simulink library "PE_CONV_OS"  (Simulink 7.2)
settings: Solver=ode45  SolverMode=SingleTasking  StartTime=0.0  StopTime=10.0  RelTol=1e-3
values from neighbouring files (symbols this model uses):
  C = 10e-3*1    (= 0.01)    [INIT_B6_2L_3Ph_IGBT_OS.m]    (also in INIT_B6_3L_3Ph_IGBT_OS.m; INIT_MMC_100L.m = 0.005; INIT_MMC_200L.m = 0.005; INIT_MMC_20L.m)
  FS = 900    [INIT_B6_2L_3Ph_IGBT_OS.m]    (also in INIT_B6_3L_3Ph_IGBT_OS.m; INIT_PWM_2L.m = 1000; INIT_PWM_3L.m = 1000; INIT_PWM_Con.m = 1000)
  LN = 2e-3    (= 0.002)    [INIT_PWM_2L.m]    (also in INIT_PWM_3L.m; INIT_PWM_Con.m; INIT_MMC_100L.m = 0.025; INIT_MMC_200L.m = 0.025)
  LS = 1e-3    (= 0.001)    [INIT_B6_2L_3Ph_IGBT_OS.m]    (also in INIT_B6_3L_3Ph_IGBT_OS.m; INIT_MMC_100L.m = 0.025; INIT_MMC_200L.m = 0.025; INIT_MMC_20L.m = 0.0025)
  LT = LN    (= 0.025)    [INIT_MMC_100L.m]    (also in INIT_MMC_200L.m; INIT_MMC_20L.m = 0.002; INIT_MMC_400L.m)
  Nc = 100    [INIT_MMC_100L.m]    (also in INIT_MMC_200L.m = 200; INIT_MMC_20L.m = 20; INIT_MMC_400L.m = 400)
  NT = sqrt(3)*340/400    [INIT_MMC_100L.m]    (also in INIT_MMC_200L.m; INIT_MMC_20L.m = sqrt(3); INIT_MMC_400L.m)
  Rg = 1e-3    (= 0.001)    [INIT_MMC_100L.m]    (also in INIT_MMC_200L.m; INIT_MMC_20L.m; INIT_MMC_400L.m)
  RN = 0.1    [INIT_PWM_2L.m]    (also in INIT_PWM_3L.m; INIT_PWM_Con.m; INIT_MMC_100L.m; INIT_MMC_200L.m)
  RT = RN    (= 0.1)    [INIT_MMC_100L.m]    (also in INIT_MMC_200L.m; INIT_MMC_20L.m; INIT_MMC_400L.m)
  UC0 = 600    [INIT_B6_2L_3Ph_IGBT_OS.m]    (also in INIT_B6_3L_3Ph_IGBT_OS.m = 500; INIT_MMC_100L.m = 6800; INIT_MMC_200L.m = 3400; INIT_MMC_20L.m = 5000)
undefined symbols (not defined in the file or in its folder): A, DT, FT, L, O1, O2, PHT, T, Td
libraries: simulink_extras x2
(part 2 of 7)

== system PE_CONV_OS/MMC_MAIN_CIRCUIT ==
  MIMC_MC_TDY_SC : S-Function  FunctionName=s_MMC_MC_TDY_SC  Parameters="[LS LN RN LT RT  NT Rg  Ron1  Ron2  Ron3]"  EnableBusSupport=off  mask(MMC_MC_TDY_SC){LS=LS, LN=LN, RN=RN, LT=LT, RT=RT, NT=NT, Rg=Rg, Ron1=1e-3, Ron2=1e-3, Ron3=1e-3}
      mask prompts: LS "LS [H]"; LN "LN [H]"; RN "RN [OHM]"; LT "LT [H]"; RT "RT [OHM]"; Rg "Rg [OHM]"; Ron1 "S1_Ron"; Ron2 "S2_Ron"; Ron3 "S3_Ron"
      mask help: Input Vector: Upper and Lower Arm Voltages =u[0...5] Grid Voltages =u[6...8] DC-Link Current =u[9] Swithing Command for Input Circuit Breaker (Antiparallel Thyristors) =u[10] Swithing Command of Short Circuit Swith (Pos. to Neg. Pass) =u[11] Swithing Command of Short Circuit Swith (Pos. to Ground) =u[12] Swithing Command of Short Circuit Swith (Neg. to Ground) =u[13] Output Vector: Upper and Lower Arm Currents =y[0...5] Converter Currents =y[6...8] Grid Currents =y[9...11] Converter Phase Voltages =y[12...14] DC-Link Voltage=y[15] Parameter Vector: Arm Inductance =p[0] Grid Inductance =p[1] Gr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
  MIMC_MC_TYD_SC : S-Function  FunctionName=s_MMC_MC_TYD_SC  Parameters="[LS LN RN LT RT  NT Rg  Ron1  Ron2  Ron3]"  EnableBusSupport=off  mask(MMC_MC_TYD_SC){LS=LS, LN=LN, RN=RN, LT=LT, RT=RT, NT=NT, Rg=Rg, Ron1=1e-3, Ron2=1e-3, Ron3=1e-3}
      mask prompts: LS "LS [H]"; LN "LN [H]"; RN "RN [OHM]"; LT "LT [H]"; RT "RT [OHM]"; Rg "Rg [OHM]"; Ron1 "S1_Ron"; Ron2 "S2_Ron"; Ron3 "S3_Ron"
      mask help: Input Vector: Upper and Lower Arm Voltages =u[0...5] Grid Voltages =u[6...8] DC-Link Current =u[9] Swithing Command for Input Circuit Breaker (Antiparallel Thyristors) =u[10] Swithing Command of Short Circuit Swith (Pos. to Neg. Pass) =u[11] Swithing Command of Short Circuit Swith (Pos. to Ground) =u[12] Swithing Command of Short Circuit Swith (Neg. to Ground) =u[13] Output Vector: Upper and Lower Arm Currents =y[0...5] Converter Currents =y[6...8] Grid Currents =y[9...11] Converter Phase Voltages =y[12...14] DC-Link Voltage=y[15] Parameter Vector: Arm Inductance =p[0] Grid Inductance =p[1] Gr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
  MIMC_MC_TYY_SC : S-Function  FunctionName=s_MMC_MC_TYY_SC  Parameters="[LS LN RN LT RT  NT Rg  Ron1  Ron2  Ron3]"  EnableBusSupport=off  mask(MMC_MC_TYY_SC){LS=LS, LN=LN, RN=RN, LT=LT, RT=RT, NT=NT, Rg=Rg, Ron1=1e-3, Ron2=1e-3, Ron3=1e-3}
      mask prompts: LS "LS [H]"; LN "LN [H]"; RN "RN [OHM]"; LT "LT [H]"; RT "RT [OHM]"; Rg "Rg [OHM]"; Ron1 "S1_Ron"; Ron2 "S2_Ron"; Ron3 "S3_Ron"
      mask help: Input Vector: Upper and Lower Arm Voltages =u[0...5] Grid Voltages =u[6...8] DC-Link Current =u[9] Swithing Command for Input Circuit Breaker (Antiparallel Thyristors) =u[10] Swithing Command of Short Circuit Swith (Pos. to Neg. Pass) =u[11] Swithing Command of Short Circuit Swith (Pos. to Ground) =u[12] Swithing Command of Short Circuit Swith (Neg. to Ground) =u[13] Output Vector: Upper and Lower Arm Currents =y[0...5] Converter Currents =y[6...8] Grid Currents =y[9...11] Converter Phase Voltages =y[12...14] DC-Link Voltage=y[15] Parameter Vector: Arm Inductance =p[0] Grid Inductance =p[1] Gr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

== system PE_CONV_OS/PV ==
  PV_Array_OS : Subsystem  mask{Isc0=7.9, Ud0=21.8, Ki=1.9e-3, Kv=-0.1, n=1.0, RS=0.28e-3*36, RP=15*36, NC=36, NMs=10, NMp=4, C=1e-3, vC0=0, RL=10000}
      mask prompts: Isc0 "Short Circuit Current at STC Isc0/Module"; Ud0 "Open Circuit Voltage at STC Ud0/Module"; Ki "Short Circuit Current Temp Coeff. Ki/Module"; Kv "Open Circuit Voltage Temp. Coeff. Kv/Module"; n "Diode Idealty Factor n"; RS "Series Resistance Rs/module "RS/Cell*NCells""; RP "Parallel Resistance RP/module "Rp/Cell*NCells""; NC "Number Cells"; NMs "Number Series Modules"; NMp "Number Parallel Modules"; C "Load Capacitor"; vC0 "init Cap Voltage"; RL "Load Res."
      mask help: PV_Array_OS with parameters: N_Cells/Module (NC), N_Series connected Module (NMs) and N_parallel connected Module (NMp) Input Vector u: u[0]=G u[1]=T u[2]=ILd Output Vector y: y[0]=PV.I y[1]=PV.V y[2]=C.I Parameter Vector p: p[0]=Isc0 p[1]=Ud0 p[2]=Ki p[3]=Kv p[4]=n p[5]=RS p[6]=RP p[7]=NC p[8]=NMs p[9]=NMp p[10]=C p[11]=vC0 p[12]=RL You can pause the simulation during running, change the Parameters you want and continue the Simulation
  P_and_O : Subsystem  mask{DeltaD=0.0001}
      mask help: MPPT controller based on the Perturb & Observe algorithm. D output = Duty cycle of the boost converter (value between 0 and 1) DeltaD = 0.0001; Increment value used to increase/decrease the duty cycle D

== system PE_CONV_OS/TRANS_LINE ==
  TL-DIST-PAR-OS : Subsystem  mask(1-Phase TL-N-DIST-PAR){L=1.3e-3, C=8.9e-9, R=0.05, TL=200, RS=50}
      mask prompts: L "L/km"; C "C/km"; R "R/km"; TL "Length[km]"
      mask help: 1 Phase frequency independent trans. Line based on the Bergerons model. Input Vector: u[0]=Input Voltage u[1]=Load Current Output Vector: y[0]=Input Voltage y[1]=Output Voltage y[2]=Input Current y[3]=Output Current PArameter Vector: p[0]= TL-Inductane L/km p[1]= TL-Capacitance C/km p[2]= TL-Resistance R/km p[3]= TL-Length [km] p[4]= TL-Input Resistance R
  TL-N-PI-3PH : Subsystem  mask(3-Phase TL N-PI-Sections){R=0.01273, L=0.9337e-3, C=12.74e-9, TL=100, N=5, RS=1, LS=1e-3}
      mask prompts: R "R/km"; L "L/km"; C "C/km"; TL "Length[km]"; N "N_Sections"
      mask help: 3 Phase trans. Line as N-PI-Sections Input Vector: u[0,1,2]=Input Voltages u[3.4]=Load Currents Output Vector: y[0,1,2]=Input Currents y[3,4,5]=Output Currents y[6,7,8]=Input Voltages y[9,10,11]=Output Voltages PArameter Vector: p[0]= TL-Resistance R/km p[1]= TL-Inductane L/km p[2]= TL-Capacitance C/km p[3]= TL-Length [km] p[4]= Number of PI-Sections N p[5]= Source-Input Resistance R
  TL-SEQ-3PH : Subsystem  mask(3-Phase TL N-Sections){R1=0.01273, R0=0.3864, L1=0.9337e-3, L0=4.1264e-3, C1=12.74e-9, C0=7.751e-9, TL=100, NS=5, RS=1, LS=1e-3}
      mask prompts: R1 "R1/km"; R0 "R0/km"; L1 "L1/km"; L0 "L0/km"; C1 "C1/km"; C0 "C0/km"; TL "Length[km]"; NS "N-Sections"
      mask help: 3 Phase trans. Line Parameters are entered as Positive and Zero Sequence Parameters Input Vector: u[0,1,2]=Input Voltages u[3,4]=Load Currents Output Vector: y[0,1,2]=Input Currents y[3,4,5]=Output Currents y[6,7,8]=Input Voltages y[9,10,11]=Output Voltages PArameter Vector: p[0]= TL-Pos. Seq. Resistance R1/km p[1]= TL-Zero Seq. Resistance R0/km p[2]= TL-Pos. Seq. Inductance L1/km p[3]= TL-Zero Seq. Inductance L0/km p[4]= TL-Pos. Seq. Capacitance C1/km p[5]= TL-Zero Seq. Capacitance C0/km p[6]= TL-Length [km] p[7]= TL-N-Sections p[8]= Source-Input Resistance RS p[9]= Source-Input Inductance LS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
  TL_N-PI_1PH : Subsystem  mask(1-Phase TL N-PI-Sections){L=1.3e-3, C=8.9e-9, R=0.05, TL=200, N=100, R1=50}
      mask prompts: L "L/km"; C "C/km"; R "R/km"; TL "Length[km]"; N "N_Sections"
      mask help: 1 Phase trans. Line as N-PI-Sections Input Vector: u[0]=Input Voltage u[1]=Load Current Output Vector: y[0]=Input Voltage y[1]=Output Voltage y[2]=Input Current y[3]=Output Current PArameter Vector: p[0]= TL-Inductane L/km p[1]= TL-Capacitance C/km p[2]= TL-Resistance R/km p[3]= TL-Length [km] p[4]= Number of PI-Sections N p[5]= TL-Input Resistance R

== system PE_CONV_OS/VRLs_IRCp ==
  IS_IRCp : Subsystem  mask(IRCp_OS){R=100, C=100e-6, VC0=0, RCs=1e-6}
      mask prompts: R "Res"; C "Cap"; VC0 "Initial Cap Voltage"; RCs "Cap Res"
      mask help: Open source IRC_Parallel Input Vector: u[0]= Is, Source Current u[1]= IL, Load Current Output Vector: y[0]=IC, Capacitance current y[1]=VC, Capacitance Voltage y[2]=VR, Resistance Voltage Parameter Vector: p[0]=R p[1]=C p[2]=VC0
  IS_IRCp_3PH : Subsystem  mask(IRCp_3PH_OS){R=100, C=100e-6, RCs=1e-6}
      mask prompts: R "Output Resistance"; C "Output Capacitance"
      mask help: Open source 3 Phase IRC_Parallel u[0,1,2]= Is1, Is2, Is3, Source Current u[3,4,5]= IL1, IL2, IL3, Load Current Output Vector: y[0,1,2]=IC_123 y[3,4,5]=VC_123 y[6,7,8]=IR_123 Parameter Vector: p[0]=R p[1]=C p[2]=RCs
  IS_VRLs : Subsystem  mask(VRLs_OS){R=1, L=10e-3, IL0=0, RLp=1e6}
      mask prompts: R "Output Resistance"; L "Output Inductance"; IL0 "Initial Inductor Current"; RLp "Ind. Parallel Res"
      mask help: Open source VRL_Series Input Vector: u[0]= Vs, Source Voltage u[1]= E, Load Voltage Output Vector: y[0]=IL, Load current y[1]=VL, Inductance Voltage y[2]=VR, Resistance Voltage Parameter Vector: p[0]=R p[1]=L p[2]=IL0 p[3]=RLp
  IS_VRLs_3PH : Subsystem  mask(VRLs_3PH_OS){R=1, L=1e-3, RLp=1e6}
      mask prompts: R "Output Resistance"; L "Output Inductance"; RLp "Ind. Parallel Res"
      mask help: Open source 3 Phase VRL_Series Input Vector: u[0,1,2]= Is1, Is2, Is3, Source Currents u[3,4,5]= E1, E2, E3, Load Voltages Output Vector: y[0,1,2]=IL1, IL2, IL3 Inductance currents y[3,4,5]=VL1, VL2, VL3 Inductance Voltages y[6,7,8]=VR1, VR2, VR3 Resistance Voltages Parameter Vector: p[0]=R p[1]=L
  VS_IRLs : Subsystem  mask(IRCp_OS){R=100}
      mask prompts: R "Res"
      mask help: Open source IRC_Parallel Input Vector: u[0]= Is, Source Current u[1]= IL, Load Current Output Vector: y[0]=IL, Load current y[1]=VL, Load Voltage Parameter Vector: p[0]=R
  VS_IRLs_3PH : Subsystem  mask(IRCp_3PH_OS){R=100}
      mask prompts: R "Output Resistance"
      mask help: Open source 3 Phase IRC_Parallel u[0,1,2]= Is1, Is2, Is3, Source Current u[3,4,5]= IL1, IL2, IL3, Load Current Output Vector: y[0,1,2]=IL_123 y[3,4,5]=VL_123 Parameter Vector: p[0]=R
  VS_VRLs : Subsystem  mask(VRLs_OS){R=1, L=10e-3, IL0=0, RLp=1e6}
      mask prompts: R "Output Resistance"; L "Output Inductance"; IL0 "Initial Inductor Current"; RLp "Ind. Parallel Res"
      mask help: Open source VRL_Series Input Vector: u[0]= Vs, Source Voltage u[1]= E, Load Voltage Output Vector: y[0]=IL, Load current y[1]=VL, Inductance Voltage y[2]=VR, Resistance Voltage Parameter Vector: p[0]=R p[1]=L p[2]=IL0
  VS_VRLs_3PH : Subsystem  mask(VRLs_3PH_OS){R=1, L=1e-3, RLp=1e6}
      mask prompts: R "Output Resistance"; L "Output Inductance"; RLp "Ind. Parallel Res"
      mask help: Open source 3 Phase VRL_Series Input Vector: u[0,1,2]= Vs1, Vs2, Vs3, Source Voltages u[3,4,5]= E1, E2, E3, Load Voltages Output Vector: y[0,1,2]=IL1, IL2, IL3 Load currents y[3,4,5]=VL1, VL2, VL3 Inductance Voltages Parameter Vector: p[0]=R p[1]=L

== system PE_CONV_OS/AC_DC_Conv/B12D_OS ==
  vS : Inport  OutDataType=sfix(16)  OutScaling=2^0
  iDC1 : Inport  Port=2  OutDataType=sfix(16)  OutScaling=2^0
  iDC2 : Inport  Port=3  OutDataType=sfix(16)  OutScaling=2^0
  Mux : Mux  Inputs="[3  1  1]"
  b12d : S-Function  FunctionName=s_b12d_OS  Parameters="[ LS  nyy  nyd   LT  LD ILD0 C  VC0  RL]"  EnableBusSupport=off
  "iD1, vD1" : Outport  OutDataType=sfix(16)  OutScaling=2^0
  "iD2, vD2" : Outport  Port=2  OutDataType=sfix(16)  OutScaling=2^0
  "iLc1, iLc2, iLc3" : Outport  Port=3  OutDataType=sfix(16)  OutScaling=2^0
  iLd1,iLd2 : Outport  Port=4  OutDataType=sfix(16)  OutScaling=2^0
  vDC1,vDC2 : Outport  Port=5  OutDataType=sfix(16)  OutScaling=2^0
  vC1,vC2 : Outport  Port=6  OutDataType=sfix(16)  OutScaling=2^0
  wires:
  b12d/6 -> vC1,vC2/1
  b12d/5 -> vDC1,vDC2/1
  iDC2/1 -> Mux/3
  b12d/3 -> "iLc1, iLc2, iLc3"/1
  b12d/1 -> "iD1, vD1"/1
  b12d/2 -> "iD2, vD2"/1
  vS/1 -> Mux/1
  iDC1/1 -> Mux/2
  Mux/1 -> b12d/1
  b12d/4 -> iLd1,iLd2/1

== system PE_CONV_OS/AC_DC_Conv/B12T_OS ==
  SWs : Inport  OutDataType=sfix(16)  OutScaling=2^0
  SWs1 : Inport  Port=2  OutDataType=sfix(16)  OutScaling=2^0
  vS : Inport  Port=3  OutDataType=sfix(16)  OutScaling=2^0
  iDC1 : Inport  Port=4  OutDataType=sfix(16)  OutScaling=2^0
  iDC2 : Inport  Port=5  OutDataType=sfix(16)  OutScaling=2^0
  Mux : Mux  Inputs="[6   6   3  1  1]"
  b12t : S-Function  FunctionName=s_b12t_OS  Parameters="[LS  LT1 LT2  LD ILD0  C  VC0 RL]"  EnableBusSupport=off
  i1T1;v1T! : Outport  OutDataType=sfix(16)  OutScaling=2^0
  i2T1,i2T1 : Outport  Port=2  OutDataType=sfix(16)  OutScaling=2^0
  "iL1, iL2, iL3" : Outport  Port=3  OutDataType=sfix(16)  OutScaling=2^0
  iDC1,iDC2 : Outport  Port=4  OutDataType=sfix(16)  OutScaling=2^0
  vDC1,vDC1 : Outport  Port=5  OutDataType=sfix(16)  OutScaling=2^0
  vC1,vC2 : Outport  Port=6  OutDataType=sfix(16)  OutScaling=2^0
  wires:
  b12t/6 -> vC1,vC2/1
  b12t/5 -> vDC1,vDC1/1
  b12t/4 -> iDC1,iDC2/1
  b12t/3 -> "iL1, iL2, iL3"/1
  iDC2/1 -> Mux/5
  SWs1/1 -> Mux/2
  SWs/1 -> Mux/1
  vS/1 -> Mux/3
  b12t/1 -> i1T1;v1T!/1
  b12t/2 -> i2T1,i2T1/1
  iDC1/1 -> Mux/4
  Mux/1 -> b12t/1

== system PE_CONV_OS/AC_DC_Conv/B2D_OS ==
  vS : Inport  OutDataType=sfix(16)  OutScaling=2^0
  iDC : Inport  Port=2  OutDataType=sfix(16)  OutScaling=2^0
  Mux : Mux  Inputs=2
  b6d : S-Function  FunctionName=s_b2d_OS  Parameters="[ LS LD  ILD0  C  VC0 RD]"  EnableBusSupport=off
  iD1,vD1 : Outport  OutDataType=sfix(16)  OutScaling=2^0
  iLc : Outport  Port=2  OutDataType=sfix(16)  OutScaling=2^0
  iLd : Outport  Port=3  OutDataType=sfix(16)  OutScaling=2^0
  vDC : Outport  Port=4  OutDataType=sfix(16)  OutScaling=2^0
  vC : Outport  Port=5  OutDataType=sfix(16)  OutScaling=2^0
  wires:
  b6d/5 -> vC/1
  b6d/4 -> vDC/1
  b6d/3 -> iLd/1
  Mux/1 -> b6d/1
  iDC/1 -> Mux/2
  vS/1 -> Mux/1
  b6d/2 -> iLc/1
  b6d/1 -> iD1,vD1/1

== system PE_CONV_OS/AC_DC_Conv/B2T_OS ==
  SWs : Inport  OutDataType=sfix(16)  OutScaling=2^0
  vS : Inport  Port=2  OutDataType=sfix(16)  OutScaling=2^0
  iDC : Inport  Port=3  OutDataType=sfix(16)  OutScaling=2^0
  Mux : Mux  Inputs="[2 1  1]"
  b6d : S-Function  FunctionName=s_b2t_OS  Parameters="[ LS LD ILD0 C  VC0 RL]"  EnableBusSupport=off
  iT1,vT1 : Outport  OutDataType=sfix(16)  OutScaling=2^0
  Ilc : Outport  Port=2  OutDataType=sfix(16)  OutScaling=2^0
  iLd : Outport  Port=3  OutDataType=sfix(16)  OutScaling=2^0
  vDC : Outport  Port=4  OutDataType=sfix(16)  OutScaling=2^0
  vC : Outport  Port=5  OutDataType=sfix(16)  OutScaling=2^0
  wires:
  b6d/5 -> vC/1
  SWs/1 -> Mux/1
  vS/1 -> Mux/2
  b6d/1 -> iT1,vT1/1
  b6d/2 -> Ilc/1
  b6d/3 -> iLd/1
  iDC/1 -> Mux/3
  Mux/1 -> b6d/1
  b6d/4 -> vDC/1

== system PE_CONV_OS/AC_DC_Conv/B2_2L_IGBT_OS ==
  SWs : Inport  OutDataType=sfix(16)  OutScaling=2^0
  vS : Inport  Port=2  OutDataType=sfix(16)  OutScaling=2^0
  iDC : Inport  Port=3  OutDataType=sfix(16)  OutScaling=2^0
  Mux : Mux  Inputs="[4  1  1]"
  b2_2L_IGBT : S-Function  FunctionName=s_b2_2L_IGBT_OS  Parameters="[ LS  C  VC0 RL]"  EnableBusSupport=off
  iT1,iD1,vT1 : Outport  OutDataType=sfix(16)  OutScaling=2^0
  iT2,iD2,vT2 : Outport  Port=2  OutDataType=sfix(16)  OutScaling=2^0
  iLs : Outport  Port=3  OutDataType=sfix(16)  OutScaling=2^0
  vDC : Outport  Port=4  OutDataType=sfix(16)  OutScaling=2^0
  va : Outport  Port=5  OutDataType=sfix(16)  OutScaling=2^0
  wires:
  b2_2L_IGBT/4 -> vDC/1
  Mux/1 -> b2_2L_IGBT/1
  iDC/1 -> Mux/3
  b2_2L_IGBT/3 -> iLs/1
  b2_2L_IGBT/2 -> iT2,iD2,vT2/1
  b2_2L_IGBT/1 -> iT1,iD1,vT1/1
  vS/1 -> Mux/2
  SWs/1 -> Mux/1
  b2_2L_IGBT/5 -> va/1

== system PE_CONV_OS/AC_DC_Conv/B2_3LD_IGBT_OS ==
  SWs : Inport  OutDataType=sfix(16)  OutScaling=2^0
  vS : Inport  Port=2  OutDataType=sfix(16)  OutScaling=2^0
  iDC : Inport  Port=3  OutDataType=sfix(16)  OutScaling=2^0
  Mux : Mux  Inputs="[8  1  1]"
  b2_2L_IGBT : S-Function  FunctionName=s_b2_3LD_IGBT_OS  Parameters="[ LS  C  VC0 RL]"  EnableBusSupport=off
  iT1,iD1,vT1 : Outport  OutDataType=sfix(16)  OutScaling=2^0
  iT2,iD2,vT2 : Outport  Port=2  OutDataType=sfix(16)  OutScaling=2^0
  iLs : Outport  Port=3  OutDataType=sfix(16)  OutScaling=2^0
  vDC12 : Outport  Port=4  OutDataType=sfix(16)  OutScaling=2^0
  va : Outport  Port=5  OutDataType=sfix(16)  OutScaling=2^0
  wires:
  b2_2L_IGBT/5 -> va/1
  SWs/1 -> Mux/1
  vS/1 -> Mux/2
  b2_2L_IGBT/1 -> iT1,iD1,vT1/1
  b2_2L_IGBT/2 -> iT2,iD2,vT2/1
  b2_2L_IGBT/3 -> iLs/1
  iDC/1 -> Mux/3
  Mux/1 -> b2_2L_IGBT/1
  b2_2L_IGBT/4 -> vDC12/1

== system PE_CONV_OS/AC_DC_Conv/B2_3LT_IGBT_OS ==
  SWs : Inport  OutDataType=sfix(16)  OutScaling=2^0
  vS : Inport  Port=2  OutDataType=sfix(16)  OutScaling=2^0
  iDC : Inport  Port=3  OutDataType=sfix(16)  OutScaling=2^0
  Mux : Mux  Inputs="[8  1  1]"
  b2_2L_IGBT : S-Function  FunctionName=s_b2_3LT_IGBT_OS  Parameters="[ LS  C  VC0 RL]"  EnableBusSupport=off
  iT1,iD1,vT1 : Outport  OutDataType=sfix(16)  OutScaling=2^0
  iT2,iD2,vT2 : Outport  Port=2  OutDataType=sfix(16)  OutScaling=2^0
  iLs : Outport  Port=3  OutDataType=sfix(16)  OutScaling=2^0
  vDC1,vDC2 : Outport  Port=4  OutDataType=sfix(16)  OutScaling=2^0
  va : Outport  Port=5  OutDataType=sfix(16)  OutScaling=2^0
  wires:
  b2_2L_IGBT/4 -> vDC1,vDC2/1
  Mux/1 -> b2_2L_IGBT/1
  iDC/1 -> Mux/3
  b2_2L_IGBT/3 -> iLs/1
  b2_2L_IGBT/2 -> iT2,iD2,vT2/1
  b2_2L_IGBT/1 -> iT1,iD1,vT1/1
  vS/1 -> Mux/2
  SWs/1 -> Mux/1
  b2_2L_IGBT/5 -> va/1

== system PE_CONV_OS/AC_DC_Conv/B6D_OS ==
  vS : Inport  OutDataType=sfix(16)  OutScaling=2^0
  iDC : Inport  Port=2  OutDataType=sfix(16)  OutScaling=2^0
  Mux : Mux  Inputs=2
  b6d : S-Function  FunctionName=s_b6d_OS  Parameters="[ LS  LD ILD0  C  VC0 RL]"  EnableBusSupport=off
  iD1,vD1 : Outport  OutDataType=sfix(16)  OutScaling=2^0
  "iLc1, iLc2, iLc3" : Outport  Port=2  OutDataType=sfix(16)  OutScaling=2^0
  iLd : Outport  Port=3  OutDataType=sfix(16)  OutScaling=2^0
  vDC : Outport  Port=4  OutDataType=sfix(16)  OutScaling=2^0
  vC : Outport  Port=5  OutDataType=sfix(16)  OutScaling=2^0
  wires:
  b6d/5 -> vC/1
  b6d/3 -> iLd/1
  b6d/2 -> "iLc1, iLc2, iLc3"/1
  b6d/4 -> vDC/1
  Mux/1 -> b6d/1
  iDC/1 -> Mux/2
  vS/1 -> Mux/1
  b6d/1 -> iD1,vD1/1

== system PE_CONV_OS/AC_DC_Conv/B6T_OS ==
  SWs : Inport  OutDataType=sfix(16)  OutScaling=2^0
  vS : Inport  Port=2  OutDataType=sfix(16)  OutScaling=2^0
  iDC : Inport  Port=3  OutDataType=sfix(16)  OutScaling=2^0
  Mux : Mux  Inputs="[6 3  1]"
  b6d : S-Function  FunctionName=s_b6t_OS  Parameters="[ LS  LD ILD0 C  VC0 RL]"  EnableBusSupport=off
  iT1,vT1 : Outport  OutDataType=sfix(16)  OutScaling=2^0
  "iLc1, iLc2, iLc3" : Outport  Port=2  OutDataType=sfix(16)  OutScaling=2^0
  iDC1 : Outport  Port=3  OutDataType=sfix(16)  OutScaling=2^0
  vDC : Outport  Port=4  OutDataType=sfix(16)  OutScaling=2^0
  vC : Outport  Port=5  OutDataType=sfix(16)  OutScaling=2^0
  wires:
  b6d/5 -> vC/1
  SWs/1 -> Mux/1
  vS/1 -> Mux/2
  b6d/1 -> iT1,vT1/1
  b6d/2 -> "iLc1, iLc2, iLc3"/1
  b6d/3 -> iDC1/1
  iDC/1 -> Mux/3
  Mux/1 -> b6d/1
  b6d/4 -> vDC/1

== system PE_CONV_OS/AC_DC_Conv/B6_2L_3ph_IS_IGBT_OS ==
  SWs : Inport  OutDataType=sfix(16)  OutScaling=2^0
  IS : Inport  Port=2  OutDataType=sfix(16)  OutScaling=2^0
  iDC : Inport  Port=3  OutDataType=sfix(16)  OutScaling=2^0
  Mux : Mux  Inputs="[6  3  1]"
  b2_IGBT : S-Function  FunctionName=s_b6_2L_3Ph_IS_IGBT_OS  Parameters="[C  UC0 RL]"  EnableBusSupport=off
  iT1,iD1,vT1 : Outport  OutDataType=sfix(16)  OutScaling=2^0
  iT2,iD2,vT2 : Outport  Port=2  OutDataType=sfix(16)  OutScaling=2^0
  vDC : Outport  Port=3  OutDataType=sfix(16)  OutScaling=2^0
  vabc : Outport  Port=4  OutDataType=sfix(16)  OutScaling=2^0
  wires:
  b2_IGBT/5 -> vabc/1
  SWs/1 -> Mux/1
  IS/1 -> Mux/2
  b2_IGBT/1 -> iT1,iD1,vT1/1
  b2_IGBT/2 -> iT2,iD2,vT2/1
  iDC/1 -> Mux/3
  Mux/1 -> b2_IGBT/1
  b2_IGBT/4 -> vDC/1

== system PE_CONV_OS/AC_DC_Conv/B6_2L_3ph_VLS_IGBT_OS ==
  SWs : Inport  OutDataType=sfix(16)  OutScaling=2^0
  vS : Inport  Port=2  OutDataType=sfix(16)  OutScaling=2^0
  iDC : Inport  Port=3  OutDataType=sfix(16)  OutScaling=2^0
  Mux : Mux  Inputs="[6  3  1]"
  b2_IGBT : S-Function  FunctionName=s_b6_2L_3Ph_VLS_IGBT_OS  Parameters="[ LS  C  UC0 RL]"  EnableBusSupport=off
  iT1,iD1,vT1 : Outport  OutDataType=sfix(16)  OutScaling=2^0
  iT2,iD2,vT2 : Outport  Port=2  OutDataType=sfix(16)  OutScaling=2^0
  iLs : Outport  Port=3  OutDataType=sfix(16)  OutScaling=2^0
  vDC : Outport  Port=4  OutDataType=sfix(16)  OutScaling=2^0
  vabc : Outport  Port=5  OutDataType=sfix(16)  OutScaling=2^0
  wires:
  b2_IGBT/4 -> vDC/1
  Mux/1 -> b2_IGBT/1
  iDC/1 -> Mux/3
  b2_IGBT/3 -> iLs/1
  b2_IGBT/2 -> iT2,iD2,vT2/1
  b2_IGBT/1 -> iT1,iD1,vT1/1
  vS/1 -> Mux/2
  SWs/1 -> Mux/1
  b2_IGBT/5 -> vabc/1

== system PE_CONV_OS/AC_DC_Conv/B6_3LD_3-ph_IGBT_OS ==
  SWs : Inport  OutDataType=sfix(16)  OutScaling=2^0
  vS : Inport  Port=2  OutDataType=sfix(16)  OutScaling=2^0
  iDC : Inport  Port=3  OutDataType=sfix(16)  OutScaling=2^0
  Mux : Mux  Inputs="[12  3  1]"
  b2_IGBT : S-Function  FunctionName=s_b6_3LD_3Ph_IGBT_OS  Parameters="[ LS  C  VC0 RL]"  EnableBusSupport=off
  iT1,iD1,vT1 : Outport  OutDataType=sfix(16)  OutScaling=2^0
  iT2,iD2,vT2 : Outport  Port=2  OutDataType=sfix(16)  OutScaling=2^0
  iLs : Outport  Port=3  OutDataType=sfix(16)  OutScaling=2^0
  vDC : Outport  Port=4  OutDataType=sfix(16)  OutScaling=2^0
  vab : Outport  Port=5  OutDataType=sfix(16)  OutScaling=2^0
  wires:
  b2_IGBT/5 -> vab/1
  SWs/1 -> Mux/1
  vS/1 -> Mux/2
  b2_IGBT/1 -> iT1,iD1,vT1/1
  b2_IGBT/2 -> iT2,iD2,vT2/1
  b2_IGBT/3 -> iLs/1
  iDC/1 -> Mux/3
  Mux/1 -> b2_IGBT/1
  b2_IGBT/4 -> vDC/1

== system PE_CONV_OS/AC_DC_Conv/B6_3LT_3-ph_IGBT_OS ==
  SWs : Inport  OutDataType=sfix(16)  OutScaling=2^0
  vS : Inport  Port=2  OutDataType=sfix(16)  OutScaling=2^0
  iDC : Inport  Port=3  OutDataType=sfix(16)  OutScaling=2^0
  Mux : Mux  Inputs="[12  3  1]"
  b2_IGBT : S-Function  FunctionName=s_b6_3LT_3Ph_IGBT_OS  Parameters="[ LS  C  VC0 RL]"  EnableBusSupport=off
  iT1,iD1,vT1 : Outport  OutDataType=sfix(16)  OutScaling=2^0
  iT2,iD2,vT2 : Outport  Port=2  OutDataType=sfix(16)  OutScaling=2^0
  iLs123 : Outport  Port=3  OutDataType=sfix(16)  OutScaling=2^0
  vDC12 : Outport  Port=4  OutDataType=sfix(16)  OutScaling=2^0
  vab : Outport  Port=5  OutDataType=sfix(16)  OutScaling=2^0
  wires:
  b2_IGBT/4 -> vDC12/1
  Mux/1 -> b2_IGBT/1
  iDC/1 -> Mux/3
  b2_IGBT/3 -> iLs123/1
  b2_IGBT/2 -> iT2,iD2,vT2/1
  b2_IGBT/1 -> iT1,iD1,vT1/1
  vS/1 -> Mux/2
  SWs/1 -> Mux/1
  b2_IGBT/5 -> vab/1

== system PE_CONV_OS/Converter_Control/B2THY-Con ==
  In1 : Inport  OutDataType=sfix(16)  OutScaling=2^0
  Mux : Mux
  THY-Con : Subsystem  mask(THY-Con){F=F, PH=PH, TD=TD}
      mask prompts: F "Frequency"; PH "Phase Angle (Degree)"; TD "Puls Duration"
      mask init:
      | x=0:pi/20:2*pi;
      | y=cos(x);
  THY-Con1 : Subsystem  mask(THY-Con){F=F, PH=-PH, TD=TD}
      mask prompts: F "Frequency"; PH "Phase Angle (Degree)"; TD "Puls Duration"
      mask init:
      | x=0:pi/20:2*pi;
      | y=cos(x);
  Out1 : Outport
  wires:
  In1/1 -> THY-Con/1(In1), THY-Con1/1(In1)
  THY-Con/1(Out1) -> Mux/1, Mux/4
  THY-Con1/1(Out1) -> Mux/2, Mux/3
  Mux/1 -> Out1/1

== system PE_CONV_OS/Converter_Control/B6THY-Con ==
  In1 : Inport  OutDataType=sfix(16)  OutScaling=2^0
  DT1 : DataTypeConversion
  Mux : Mux  Inputs=6
  OR{,1..5} (6 alike) : Logic  Operator=OR
  THY-Con : Subsystem  mask(THY-Con){F=F, PH=PH, TD=TD}
      mask prompts: F "Frequency"; PH "Phase Angle (Degree)"; TD "Puls Duration"
      mask init:
      | x=0:pi/20:2*pi;
      | y=cos(x);
  THY-Con1 : Subsystem  mask(THY-Con){F=F, PH=PH-60, TD=TD}
      mask prompts: F "Frequency"; PH "Phase Angle (Degree)"; TD "Puls Duration"
      mask init:
      | x=0:pi/20:2*pi;
      | y=cos(x);
  THY-Con2 : Subsystem  mask(THY-Con){F=F, PH=PH-120, TD=TD}
      mask prompts: F "Frequency"; PH "Phase Angle (Degree)"; TD "Puls Duration"
      mask init:
      | x=0:pi/20:2*pi;
      | y=cos(x);
  THY-Con3 : Subsystem  mask(THY-Con){F=F, PH=PH-180, TD=TD}
      mask prompts: F "Frequency"; PH "Phase Angle (Degree)"; TD "Puls Duration"
      mask init:
      | x=0:pi/20:2*pi;
      | y=cos(x);
  THY-Con4 : Subsystem  mask(THY-Con){F=F, PH=PH-240, TD=TD}
      mask prompts: F "Frequency"; PH "Phase Angle (Degree)"; TD "Puls Duration"
      mask init:
      | x=0:pi/20:2*pi;
      | y=cos(x);
  THY-Con5 : Subsystem  mask(THY-Con){F=F, PH=PH-300, TD=TD}
      mask prompts: F "Frequency"; PH "Phase Angle (Degree)"; TD "Puls Duration"
      mask init:
      | x=0:pi/20:2*pi;
      | y=cos(x);
  Out1 : Outport
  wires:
  OR5/1 -> Mux/6
  OR4/1 -> Mux/5
  OR3/1 -> Mux/4
  OR2/1 -> Mux/3
  OR1/1 -> Mux/2
  OR/1 -> Mux/1
  THY-Con/1(Out1) -> OR5/2, OR/1
  THY-Con5/1(Out1) -> OR4/2, OR5/1
  THY-Con4/1(Out1) -> OR3/2, OR4/1
  THY-Con3/1(Out1) -> OR2/2, OR3/1
  THY-Con2/1(Out1) -> OR1/2, OR2/1
  THY-Con1/1(Out1) -> OR/2, OR1/1
  Mux/1 -> DT1/1
  In1/1 -> THY-Con4/1(In1), THY-Con5/1(In1), THY-Con3/1(In1), THY-Con2/1(In1), THY-Con1/1(In1), THY-Con/1(In1)
  DT1/1 -> Out1/1

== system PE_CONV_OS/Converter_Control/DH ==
  I : Inport  OutDataType=sfix(16)  OutScaling=2^0
  Gain : Gain  Gain=1/2  ParameterDataType=sfix(16)  ParameterScaling=2^0  OutDataType=sfix(16)  OutScaling=2^0
  MinMax : MinMax  OutDataType=sfix(16)  OutScaling=2^0
  MinMax1 : MinMax  Function=max  OutDataType=sfix(16)  OutScaling=2^0
  Sum6 : Sum  Inputs=--  OutDataType=sfix(16)  OutScaling=2^0
  Sum7 : Sum  OutDataType=sfix(16)  OutScaling=2^0
  O : Outport  InitialOutput=0
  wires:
  I/1 -> MinMax1/1, MinMax/1, Sum7/1
  MinMax/1 -> Sum6/1
  MinMax1/1 -> Sum6/2
  Sum6/1 -> Gain/1
  Gain/1 -> Sum7/2
  Sum7/1 -> O/1

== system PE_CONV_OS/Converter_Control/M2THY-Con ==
  In1 : Inport  OutDataType=sfix(16)  OutScaling=2^0
  Mux : Mux  Inputs=2
  THY-Con : Subsystem  mask(THY-Con){F=F, PH=PH, TD=TD}
      mask prompts: F "Frequency"; PH "Phase Angle (Degree)"; TD "Puls Duration"
      mask init:
      | x=0:pi/20:2*pi;
      | y=cos(x);
  THY-Con1 : Subsystem  mask(THY-Con){F=F, PH=-PH, TD=TD}
      mask prompts: F "Frequency"; PH "Phase Angle (Degree)"; TD "Puls Duration"
      mask init:
      | x=0:pi/20:2*pi;
      | y=cos(x);
  Out1 : Outport
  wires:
  Mux/1 -> Out1/1
  THY-Con/1(Out1) -> Mux/1
  THY-Con1/1(Out1) -> Mux/2
  In1/1 -> THY-Con/1(In1), THY-Con1/1(In1)

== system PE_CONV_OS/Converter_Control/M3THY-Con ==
  In1 : Inport  OutDataType=sfix(16)  OutScaling=2^0
  Mux : Mux  Inputs=3
  THY-Con : Subsystem  mask(THY-Con){F=F, PH=PH, TD=TD}
      mask prompts: F "Frequency"; PH "Phase Angle (Degree)"; TD "Puls Duration"
      mask init:
      | x=0:pi/20:2*pi;
      | y=cos(x);
  THY-Con1 : Subsystem  mask(THY-Con){F=F, PH=PH-120, TD=TD}
      mask prompts: F "Frequency"; PH "Phase Angle (Degree)"; TD "Puls Duration"
      mask init:
      | x=0:pi/20:2*pi;
      | y=cos(x);
  THY-Con2 : Subsystem  mask(THY-Con){F=F, PH=PH-240, TD=TD}
      mask prompts: F "Frequency"; PH "Phase Angle (Degree)"; TD "Puls Duration"
      mask init:
      | x=0:pi/20:2*pi;
      | y=cos(x);
  Out1 : Outport
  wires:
  In1/1 -> THY-Con1/1(In1), THY-Con2/1(In1), THY-Con/1(In1)
  THY-Con2/1(Out1) -> Mux/3
  THY-Con1/1(Out1) -> Mux/2
  THY-Con/1(Out1) -> Mux/1
  Mux/1 -> Out1/1

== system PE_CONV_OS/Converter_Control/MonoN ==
  s1 : Inport  OutDataType=sfix(16)  OutScaling=2^0
  Constant : Constant  OutDataType=sfix(16)  OutScaling=2^0
  DT{,1..3} (4 alike) : DataTypeConversion
  Int : Integrator  ExternalReset=falling
  J-K Flip-Flop : simulink_extras/Flip Flops/J-K Flip-Flop  initial_condition=0
  Logical Operator : Logic
  Rel1 : Relay  OnSwitchValue=PW  OnOutputValue=0  OffOutputValue=1  OutDataType=sfix(16)  OutScaling=2^0
  Terminator : Terminator
  not : Logic  Operator=NOT
  s1d : Outport  InitialOutput=0
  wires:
  not/1 -> J-K Flip-Flop/3
  Constant/1 -> DT3/1
  s1/1 -> DT2/1, Int/2
  Logical Operator/1 -> DT1/1
  J-K Flip-Flop/1 -> Logical Operator/1, DT/1
  Rel1/1 -> Logical Operator/2
  J-K Flip-Flop/2 -> Terminator/1
  Int/1 -> Rel1/1
  DT/1 -> Int/1
  DT1/1 -> s1d/1
  DT2/1 -> J-K Flip-Flop/2
  DT3/1 -> J-K Flip-Flop/1, not/1

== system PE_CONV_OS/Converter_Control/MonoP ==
  s1 : Inport  OutDataType=sfix(16)  OutScaling=2^0
  Constant : Constant  OutDataType=sfix(16)  OutScaling=2^0
  D Latch : simulink_extras/Flip Flops/D Latch  SystemSampleTime=-1
  DT{,1..5} (6 alike) : DataTypeConversion
  Int : Integrator  ExternalReset=rising
  Logical Operator : Logic
  Rel1 : Relay  OnSwitchValue=PW  OnOutputValue=0  OffOutputValue=1  OutDataType=sfix(16)  OutScaling=2^0
  Terminator : Terminator
  s1d : Outport  InitialOutput=0
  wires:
  D Latch/2 -> Terminator/1
  Rel1/1 -> DT4/1
  D Latch/1 -> DT/1, DT3/1
  s1/1 -> DT2/1, Int/2
  Constant/1 -> DT5/1
  Logical Operator/1 -> DT1/1
  Int/1 -> Rel1/1
  DT/1 -> Int/1
  DT1/1 -> s1d/1
  DT2/1 -> D Latch/2
  DT3/1 -> Logical Operator/1
  DT4/1 -> Logical Operator/2
  DT5/1 -> D Latch/1

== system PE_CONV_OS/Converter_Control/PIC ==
  c* : Inport  OutDataType=sfix(16)  OutScaling=2^0
  c : Inport  Port=2  OutDataType=sfix(16)  OutScaling=2^0
  Gain : Gain  Gain=Ki  ParameterDataType=sfix(16)  ParameterScaling=2^0  OutDataType=sfix(16)  OutScaling=2^0
  Gain1 : Gain  Gain=Kp  ParameterDataType=sfix(16)  ParameterScaling=2^0  OutDataType=sfix(16)  OutScaling=2^0
  Integrator : Integrator  UpperSaturationLimit=lim  LowerSaturationLimit=-lim
  Saturation : Saturate  UpperLimit=lim  LowerLimit=-lim
  Sum1 : Sum  Inputs=+-  OutDataType=sfix(16)  OutScaling=2^0
  Sum2 : Sum  OutDataType=sfix(16)  OutScaling=2^0
  e* : Outport  InitialOutput=0
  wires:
  Gain/1 -> Integrator/1
  Gain1/1 -> Sum2/1
  Sum1/1 -> Gain/1, Gain1/1
  Sum2/1 -> Saturation/1
  Saturation/1 -> e*/1
  c/1 -> Sum1/2
  c*/1 -> Sum1/1
  Integrator/1 -> Sum2/2

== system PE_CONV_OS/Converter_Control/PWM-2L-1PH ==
  In1 : Inport  OutDataType=sfix(16)  OutScaling=2^0
  DT : DataTypeConversion
  DT1 : DataTypeConversion
  Mux : Mux  Inputs=2
  Relay : Relay  OutDataType=sfix(16)  OutScaling=2^0
  Sum : Sum  Inputs=+-  OutDataType=sfix(16)  OutScaling=2^0
  TonDelay : Subsystem  mask(TonDelay){DT=DT}
      mask prompts: DT "Dead Time"
      mask help: Turn on dead time to protect against short circuit of the converter leg
  TonDelay1 : Subsystem  mask(TonDelay){DT=DT}
      mask prompts: DT "Dead Time"
      mask help: Turn on dead time to protect against short circuit of the converter leg
  TriGtr : Subsystem  mask(TriGtr){T=1/FT, Td=PHT/FT/360}
      mask prompts: T "Period Time"; Td "Time Delay"
      mask help: Triangular Wave Generator with variable time delay
  not : Logic  Operator=NOT  Inputs=1
  Out1 : Outport  InitialOutput=0
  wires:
  Mux/1 -> Out1/1
  TonDelay/1(s1d) -> Mux/1
  Relay/1 -> TonDelay/1(s1), DT1/1
  TonDelay1/1(s1d) -> Mux/2
  not/1 -> DT/1
  Sum/1 -> Relay/1
  TriGtr/1(O) -> Sum/2
  In1/1 -> Sum/1
  DT/1 -> TonDelay1/1(s1)
  DT1/1 -> not/1

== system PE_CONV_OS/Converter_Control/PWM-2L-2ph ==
  I1 : Inport  OutDataType=sfix(16)  OutScaling=2^0
  Gain : Gain  Gain=-1  ParameterDataType=sfix(16)  ParameterScaling=2^0  OutDataType=sfix(16)  OutScaling=2^0
  Mux : Mux  Inputs=2
  PWM-2L-1PH : Subsystem  mask(PWM-2L-1PH){FT=FT, PHT=PHT, DT=DT}
      mask prompts: FT "Triangular Frequency"; PHT "Trian. Phase Angle (Degree)"; DT "Dead Time"
      mask help: Pulse Width Modulation for 1 Phase Converter
  PWM-2L-1PH1 : Subsystem  mask(PWM-2L-1PH){FT=FT, PHT=PHT, DT=DT}
      mask prompts: FT "Triangular Frequency"; PHT "Trian. Phase Angle (Degree)"; DT "Dead Time"
      mask help: Pulse Width Modulation for 1 Phase Converter
  O1 : Outport
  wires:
  Mux/1 -> O1/1
  PWM-2L-1PH1/1(Out1) -> Mux/2
  PWM-2L-1PH/1(Out1) -> Mux/1
  I1/1 -> PWM-2L-1PH/1(In1), Gain/1
  Gain/1 -> PWM-2L-1PH1/1(In1)

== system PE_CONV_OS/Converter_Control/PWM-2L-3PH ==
  In4 : Inport  OutDataType=sfix(16)  OutScaling=2^0
  Demux : Demux  Outputs=3
  Mux : Mux  Inputs=3
  PWM-2L-1PH : Subsystem  mask(PWM-2L-1PH){FT=FT, PHT=PHT, DT=DT}
      mask prompts: FT "Triangular Frequency"; PHT "Trian. Phase Angle (Degree)"; DT "Dead Time"
      mask help: Pulse Width Modulation for 1 Phase Converter
  PWM-2L-1PH1 : Subsystem  mask(PWM-2L-1PH){FT=FT, PHT=PHT, DT=DT}
      mask prompts: FT "Triangular Frequency"; PHT "Trian. Phase Angle (Degree)"; DT "Dead Time"
      mask help: Pulse Width Modulation for 1 Phase Converter
  PWM-2L-1PH2 : Subsystem  mask(PWM-2L-1PH){FT=FT, PHT=PHT, DT=DT}
      mask prompts: FT "Triangular Frequency"; PHT "Trian. Phase Angle (Degree)"; DT "Dead Time"
      mask help: Pulse Width Modulation for 1 Phase Converter
  Out1 : Outport
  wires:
  Mux/1 -> Out1/1
  PWM-2L-1PH2/1(Out1) -> Mux/3
  PWM-2L-1PH/1(Out1) -> Mux/1
  PWM-2L-1PH1/1(Out1) -> Mux/2
  Demux/1 -> PWM-2L-1PH/1(In1)
  Demux/2 -> PWM-2L-1PH1/1(In1)
  Demux/3 -> PWM-2L-1PH2/1(In1)
  In4/1 -> Demux/1

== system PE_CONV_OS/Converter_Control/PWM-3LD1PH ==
  In1 : Inport  OutDataType=sfix(16)  OutScaling=2^0
  Mux : Mux
  SS : Subsystem
  SS1 : Subsystem
  Out1 : Outport
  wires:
  In1/1 -> SS1/1(I1), SS/1(I1)
  SS1/1(O1) -> Mux/2
  SS/2(O2) -> Mux/3
  Mux/1 -> Out1/1
  SS/1(O1) -> Mux/1
  SS1/2(O2) -> Mux/4

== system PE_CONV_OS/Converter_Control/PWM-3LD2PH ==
  In1 : Inport  OutDataType=sfix(16)  OutScaling=2^0
  Gain : Gain  Gain=-1  ParameterDataType=sfix(16)  ParameterScaling=2^0  OutDataType=sfix(16)  OutScaling=2^0
  Mux1 : Mux  Inputs=2
  PWM-3LD1PH : Subsystem  mask(PWM-3LD1PH){FT=FT, PHT=PHT, A=A, O1=O1, O2=O2, DT=DT}
      mask prompts: FT "Frequency of Trian Sig."; PHT "Phase Angle of Trian. Sig."; A "Amplitude of Trian. Sig."; O1 "Offset of 1st Trian"; O2 "Offset of 2nd Trian."; DT "Dead Time"
      mask help: Pulse Width Modulation for 1 Phase 3 Level Floating Capacitor Converter
  PWM-3LD1PH1 : Subsystem  mask(PWM-3LD1PH){FT=FT, PHT=PHT, A=A, O1=O1, O2=O2, DT=DT}
      mask prompts: FT "Frequency of Trian Sig."; PHT "Phase Angle of Trian. Sig."; A "Amplitude of Trian. Sig."; O1 "Offset of 1st Trian"; O2 "Offset of 2nd Trian."; DT "Dead Time"
      mask help: Pulse Width Modulation for 1 Phase 3 Level Floating Capacitor Converter
  Out1 : Outport
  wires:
  Mux1/1 -> Out1/1
  Gain/1 -> PWM-3LD1PH1/1(In1)
  In1/1 -> PWM-3LD1PH/1(In1), Gain/1
  PWM-3LD1PH/1(Out1) -> Mux1/1
  PWM-3LD1PH1/1(Out1) -> Mux1/2

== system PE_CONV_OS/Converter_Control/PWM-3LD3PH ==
  In1 : Inport  OutDataType=sfix(16)  OutScaling=2^0
  Demux1 : Demux  Outputs=3
  Mux1 : Mux  Inputs=3
  PWM-3LD1PH : Subsystem  mask(PWM-3LD_1PH){FT=FT, PHT=PHT, A=A, O1=O1, O2=O2, DT=DT}
      mask prompts: FT "Frequency of Trian Sig."; PHT "Phase Angle of Trian. Sig."; A "Amplitude of Trian. Sig."; O1 "Offset of 1st Trian"; O2 "Offset of 2nd Trian."; DT "Dead Time"
      mask help: Pulse Width Modulation for 1 Leg of 3 Level Neutral point clamped Converter
  PWM-3LD1PH1 : Subsystem  mask(PWM-3LD_1PH){FT=FT, PHT=PHT, A=A, O1=O1, O2=O2, DT=DT}
      mask prompts: FT "Frequency of Trian Sig."; PHT "Phase Angle of Trian. Sig."; A "Amplitude of Trian. Sig."; O1 "Offset of 1st Trian"; O2 "Offset of 2nd Trian."; DT "Dead Time"
      mask help: Pulse Width Modulation for 1 Leg of 3 Level Neutral point clamped Converter
  PWM-3LD1PH2 : Subsystem  mask(PWM-3LD_1PH){FT=FT, PHT=PHT, A=A, O1=O1, O2=O2, DT=DT}
      mask prompts: FT "Frequency of Trian Sig."; PHT "Phase Angle of Trian. Sig."; A "Amplitude of Trian. Sig."; O1 "Offset of 1st Trian"; O2 "Offset of 2nd Trian."; DT "Dead Time"
      mask help: Pulse Width Modulation for 1 Leg of 3 Level Neutral point clamped Converter
  Out1 : Outport
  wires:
  PWM-3LD1PH/1(Out1) -> Mux1/1
  PWM-3LD1PH1/1(Out1) -> Mux1/2
  PWM-3LD1PH2/1(Out1) -> Mux1/3
  Mux1/1 -> Out1/1
  Demux1/1 -> PWM-3LD1PH/1(In1)
  Demux1/2 -> PWM-3LD1PH1/1(In1)
  Demux1/3 -> PWM-3LD1PH2/1(In1)
  In1/1 -> Demux1/1

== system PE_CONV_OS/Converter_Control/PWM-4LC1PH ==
  In1 : Inport  OutDataType=sfix(16)  OutScaling=2^0
  Mux : Mux  Inputs=6
  PWM-2L-1PH : Subsystem  mask(PWM-2L-1PH){FT=FT, PHT=PHT1, DT=DT}
      mask prompts: FT "Triangular Frequency"; PHT "Trian. Phase Angle (Degree)"; DT "Dead Time"
      mask help: Pulse Width Modulation for 1 Phase Converter
  PWM-2L-1PH1 : Subsystem  mask(PWM-2L-1PH){FT=FT, PHT=PHT2, DT=DT}
      mask prompts: FT "Triangular Frequency"; PHT "Trian. Phase Angle (Degree)"; DT "Dead Time"
      mask help: Pulse Width Modulation for 1 Phase Converter
  PWM-2L-1PH2 : Subsystem  mask(PWM-2L-1PH){FT=FT, PHT=PHT3, DT=DT}
      mask prompts: FT "Triangular Frequency"; PHT "Trian. Phase Angle (Degree)"; DT "Dead Time"
      mask help: Pulse Width Modulation for 1 Phase Converter
  Out1 : Outport
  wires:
  PWM-2L-1PH/2(Out2) -> Mux/6
  In1/1 -> PWM-2L-1PH2/1(In1), PWM-2L-1PH1/1(In1), PWM-2L-1PH/1(In1)
  Mux/1 -> Out1/1
  PWM-2L-1PH2/2(Out2) -> Mux/4
  PWM-2L-1PH2/1(Out1) -> Mux/3
  PWM-2L-1PH1/2(Out2) -> Mux/5
  PWM-2L-1PH1/1(Out1) -> Mux/2
  PWM-2L-1PH/1(Out1) -> Mux/1

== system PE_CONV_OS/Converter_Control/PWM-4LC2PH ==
  In1 : Inport  OutDataType=sfix(16)  OutScaling=2^0
  Gain : Gain  Gain=-1  ParameterDataType=sfix(16)  ParameterScaling=2^0  OutDataType=sfix(16)  OutScaling=2^0
  Mux : Mux  Inputs=2
  PWM-4LC1PH : Subsystem  mask(PWM-4LC1PH){FT=900, PHT1=0, PHT2=-120, PHT3=-240, DT=1e-6}
      mask prompts: FT "Frequency of Trian Sig."; PHT1 "Phase Angle of 1st Trian. Sig."; PHT2 "Phase Angle of 2nd Trian. Sig."; PHT3 "Phase Angle of 3rd Trian. Sig."; DT "Dead Time"
      mask help: Pulse Width Modulation for 1 Phase 4 Level Floating Capacitor Converter
  PWM-4LC1PH1 : Subsystem  mask(PWM-4LC1PH){FT=900, PHT1=0, PHT2=-120, PHT3=-240, DT=1e-6}
      mask prompts: FT "Frequency of Trian Sig."; PHT1 "Phase Angle of 1st Trian. Sig."; PHT2 "Phase Angle of 2nd Trian. Sig."; PHT3 "Phase Angle of 3rd Trian. Sig."; DT "Dead Time"
      mask help: Pulse Width Modulation for 1 Phase 4 Level Floating Capacitor Converter
  Out1 : Outport
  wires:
  Gain/1 -> PWM-4LC1PH1/1(In1)
  Mux/1 -> Out1/1
  PWM-4LC1PH/1(Out1) -> Mux/1
  PWM-4LC1PH1/1(Out1) -> Mux/2
  In1/1 -> Gain/1, PWM-4LC1PH/1(In1)

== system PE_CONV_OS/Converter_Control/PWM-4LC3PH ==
  In1 : Inport  OutDataType=sfix(16)  OutScaling=2^0
  Demux : Demux  Outputs=3
  Mux : Mux  Inputs=3
  PWM-4LC1PH : Subsystem  mask(PWM-4LC1PH){FT=FT, PHT1=PHT1, PHT2=PHT2, PHT3=PHT3, DT=DT}
      mask prompts: FT "Frequency of Trian Sig."; PHT1 "Phase Angle of 1st Trian. Sig."; PHT2 "Phase Angle of 2nd Trian. Sig."; PHT3 "Phase Angle of 3rd Trian. Sig."; DT "Dead Time"
      mask help: Pulse Width Modulation for 1 Phase 4 Level Floating Capacitor Converter
  PWM-4LC1PH1 : Subsystem  mask(PWM-4LC1PH){FT=FT, PHT1=PHT1, PHT2=PHT2, PHT3=PHT3, DT=DT}
      mask prompts: FT "Frequency of Trian Sig."; PHT1 "Phase Angle of 1st Trian. Sig."; PHT2 "Phase Angle of 2nd Trian. Sig."; PHT3 "Phase Angle of 3rd Trian. Sig."; DT "Dead Time"
      mask help: Pulse Width Modulation for 1 Phase 4 Level Floating Capacitor Converter
  PWM-4LC1PH2 : Subsystem  mask(PWM-4LC1PH){FT=FT, PHT1=PHT1, PHT2=PHT2, PHT3=PHT3, DT=DT}
      mask prompts: FT "Frequency of Trian Sig."; PHT1 "Phase Angle of 1st Trian. Sig."; PHT2 "Phase Angle of 2nd Trian. Sig."; PHT3 "Phase Angle of 3rd Trian. Sig."; DT "Dead Time"
      mask help: Pulse Width Modulation for 1 Phase 4 Level Floating Capacitor Converter
  Out1 : Outport
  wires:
  In1/1 -> Demux/1
  Mux/1 -> Out1/1
  Demux/3 -> PWM-4LC1PH2/1(In1)
  Demux/2 -> PWM-4LC1PH1/1(In1)
  Demux/1 -> PWM-4LC1PH/1(In1)
  PWM-4LC1PH2/1(Out1) -> Mux/3
  PWM-4LC1PH1/1(Out1) -> Mux/2
  PWM-4LC1PH/1(Out1) -> Mux/1

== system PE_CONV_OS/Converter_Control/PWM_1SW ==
  In1 : Inport  OutDataType=sfix(16)  OutScaling=2^0
  Relay : Relay  OutDataType=sfix(16)  OutScaling=2^0
  SoToG1 : Subsystem  mask(SoToG){T=1/FS}
      mask prompts: T "Period Time"
      mask help: Saw tooth Generator Input: Period Time
  Sum : Sum  Inputs=+-  OutDataType=sfix(16)  OutScaling=2^0
  Out1 : Outport  InitialOutput=0
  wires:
  Sum/1 -> Relay/1
  In1/1 -> Sum/1
  SoToG1/1(O) -> Sum/2
  Relay/1 -> Out1/1

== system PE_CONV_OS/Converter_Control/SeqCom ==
  abc : Inport  OutDataType=sfix(16)  OutScaling=2^0
  NegSeq : Subsystem
  PosSeq : Subsystem
  ZeroSeq : Subsystem
  Pos : Outport
  Neg : Outport  Port=2
  Zero : Outport  Port=3
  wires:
  ZeroSeq/1(Out1) -> Zero/1
  NegSeq/1(Out1) -> Neg/1
  PosSeq/1(Out1) -> Pos/1
  abc/1 -> NegSeq/1(In1), ZeroSeq/1(In1), PosSeq/1(In1)

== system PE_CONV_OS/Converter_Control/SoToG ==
  Clock : Clock
  P : Product  OutDataType=sfix(16)  OutScaling=2^0
  T1 : Constant  Value=T  OutDataType=sfix(16)  OutScaling=2^0
  T2 : Constant  Value=1/T  OutDataType=sfix(16)  OutScaling=2^0
  mod : Math  Operator=mod
  O : Outport
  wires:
  P/1 -> O/1
  mod/1 -> P/1
  T2/1 -> P/2
  T1/1 -> mod/2
  Clock/1 -> mod/1

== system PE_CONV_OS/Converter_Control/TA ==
  Ampl. : Gain  Gain=A
  Offset : Constant  Value=O
  Sum : Sum
  TG : S-Function  FunctionName=TG_MMC  Parameters=[Nc, T]  EnableBusSupport=off
  Out1 : Outport
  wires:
  TG/1 -> Ampl./1
  Sum/1 -> Out1/1
  Ampl./1 -> Sum/1
  Offset/1 -> Sum/2

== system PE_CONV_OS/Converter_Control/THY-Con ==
  In1 : Inport  OutDataType=sfix(16)  OutScaling=2^0
  DT : DataTypeConversion
  DT1 : DataTypeConversion
  DT2 : DataTypeConversion
  Fcn : Fcn  Expr="(u  > 0.9999)*2 + (u<=0.9999)*u"
  Relay : Relay  OutDataType=sfix(16)  OutScaling=2^0
  Sine Wave1 : Sin  Frequency=F*2*pi  Phase=PH*pi/180  SampleTime=0
  Sum1 : Sum  Inputs=-+  OutDataType=sfix(16)  OutScaling=2^0
  TonDelay : Subsystem  mask(TonDelay){DT=TD}
      mask prompts: DT "Dead Time"
      mask help: Turn on dead time to protect against short circuit of the converter leg
  XOR : Logic  Operator=XOR
  Out1 : Outport
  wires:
  Fcn/1 -> Sum1/1
  Sine Wave1/1 -> Fcn/1
  XOR/1 -> DT/1
  Relay/1 -> TonDelay/1(s1), DT2/1
  TonDelay/1(s1d) -> DT1/1
  Sum1/1 -> Relay/1
  In1/1 -> Sum1/2
  DT/1 -> Out1/1
  DT1/1 -> XOR/1
  DT2/1 -> XOR/2

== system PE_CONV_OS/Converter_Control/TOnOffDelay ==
  In1 : Inport  OutDataType=sfix(16)  OutScaling=2^0
  DT : DataTypeConversion
  Int : Integrator  ExternalReset=rising
  N1 : Logic  Operator=NOT
  Rel1 : Relay  OnSwitchValue=DT_ON  OutDataType=sfix(16)  OutScaling=2^0
  TonDelay : Subsystem  mask(TonDelay){DT=DT_OFF}
      mask prompts: DT "Dead Time"
      mask help: Turn on dead time to protect against short circuit of the converter leg
  Out1 : Outport
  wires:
  N1/1 -> DT/1
  Int/1 -> Rel1/1
  In1/1 -> Int/1, N1/1
  TonDelay/1(s1d) -> Int/2
  Rel1/1 -> Out1/1
  DT/1 -> TonDelay/1(s1)

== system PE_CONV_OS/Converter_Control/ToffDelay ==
  In1 : Inport  OutDataType=sfix(16)  OutScaling=2^0
  DT : DataTypeConversion
  DT1 : DataTypeConversion
  DT2 : DataTypeConversion
  N1 : Logic  Operator=NOT
  N2 : Logic  Operator=NOT
  TonDelay : Subsystem  mask(TonDelay){DT=DT}
      mask prompts: DT "Dead Time"
      mask help: Turn on dead time to protect against short circuit of the converter leg
  Out1 : Outport
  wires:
  N2/1 -> DT/1
  TonDelay/1(s1d) -> DT2/1
  In1/1 -> N1/1
  N1/1 -> DT1/1
  DT/1 -> Out1/1
  DT1/1 -> TonDelay/1(s1)
  DT2/1 -> N2/1

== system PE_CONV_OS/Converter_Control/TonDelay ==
  s1 : Inport  Orientation=down  OutDataType=sfix(16)  OutScaling=2^0
  Int : Integrator  ExternalReset=falling
  Rel1 : Relay  OnSwitchValue=DT  OutDataType=sfix(16)  OutScaling=2^0
  s1d : Outport  InitialOutput=0
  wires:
  Rel1/1 -> s1d/1
  s1/1 -> Int/1, Int/2
  Int/1 -> Rel1/1

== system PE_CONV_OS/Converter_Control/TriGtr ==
  Clock : Clock
  Fcn : Fcn  Expr="(u* (u <=T/4) * 4/T)   +  (  (u > T/4) && ( u <=3*T/4) )* ( 1 - (u-T/4) *4/T )   +  ( (u > 3*T/4)&& (u<=T)) * ( ((u -3*T/4)* 4/T )-1 )"
  Sum : Sum
  T : Constant  Value=T
  Td : Constant  Value=Td
  mod : Math  Operator=mod
  O : Outport  InitialOutput=0
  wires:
  mod/1 -> Fcn/1
  Fcn/1 -> O/1
  Clock/1 -> Sum/1
  T/1 -> mod/2
  Sum/1 -> mod/1
  Td/1 -> Sum/2

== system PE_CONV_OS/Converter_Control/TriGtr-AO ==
  Ampl. : Gain  Gain=A
  Offset : Constant  Value=O
  Sum : Sum
  TriGtr : Subsystem  mask(TriGtr){T=T, Td=Td}
      mask prompts: T "Period Time"; Td "Time Delay"
      mask help: Triangular Wave Generator with variable time delay
  Out1 : Outport
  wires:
  Sum/1 -> Out1/1
  Ampl./1 -> Sum/1
  TriGtr/1(O) -> Ampl./1
  Offset/1 -> Sum/2

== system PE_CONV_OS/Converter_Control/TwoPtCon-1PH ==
  Iref : Inport  OutDataType=sfix(16)  OutScaling=2^0
  Iact : Inport  Port=2  OutDataType=sfix(16)  OutScaling=2^0
  DT : DataTypeConversion
  DT1 : DataTypeConversion
  Mux : Mux  Inputs=2
  Relay : Relay  OnSwitchValue=SP  OffSwitchValue=SN  OutDataType=sfix(16)  OutScaling=2^0
  Sum : Sum  Inputs=+-  OutDataType=sfix(16)  OutScaling=2^0
  TonDelay : Subsystem  mask(TonDelay){DT=DT}
      mask prompts: DT "Dead Time"
      mask help: Turn on dead time to protect against short circuit of the converter leg
  TonDelay1 : Subsystem  mask(TonDelay){DT=DT}
      mask prompts: DT "Dead Time"
      mask help: Turn on dead time to protect against short circuit of the converter leg
  not : Logic  Operator=NOT  Inputs=1
  S1 : Outport  InitialOutput=0
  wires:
  Mux/1 -> S1/1
  TonDelay/1(s1d) -> Mux/1
  TonDelay1/1(s1d) -> Mux/2
  Relay/1 -> TonDelay/1(s1), DT1/1
  not/1 -> DT/1
  Sum/1 -> Relay/1
  Iact/1 -> Sum/2
  Iref/1 -> Sum/1
  DT/1 -> TonDelay1/1(s1)
  DT1/1 -> not/1

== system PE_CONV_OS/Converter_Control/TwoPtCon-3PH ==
  Iref : Inport  OutDataType=sfix(16)  OutScaling=2^0
  Iact : Inport  Port=2  OutDataType=sfix(16)  OutScaling=2^0
  Demux : Demux  Outputs=3
  Demux1 : Demux  Outputs=3
  Mux : Mux  Inputs=6
  TwoPtCon-1Ph : Subsystem  mask(TwoPtCon-1Ph){SP=SP, SN=SN, DT=DT}
      mask prompts: SP "Positive Limit"; SN "Negative Limit"; DT "Dead Time"
      mask help: Two Point Controller with Dead Time protection for 1Phase Converter
  TwoPtCon-1Ph1 : Subsystem  mask(TwoPtCon-1Ph){SP=SP, SN=SN, DT=DT}
      mask prompts: SP "Positive Limit"; SN "Negative Limit"; DT "Dead Time"
      mask help: Two Point Controller with Dead Time protection for 1Phase Converter
  TwoPtCon-1Ph2 : Subsystem  mask(TwoPtCon-1Ph){SP=SP, SN=SN, DT=DT}
      mask prompts: SP "Positive Limit"; SN "Negative Limit"; DT "Dead Time"
      mask help: Two Point Controller with Dead Time protection for 1Phase Converter
  s05 : Outport
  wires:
  TwoPtCon-1Ph2/2(Out2) -> Mux/6
  TwoPtCon-1Ph2/1(Out1) -> Mux/5
  TwoPtCon-1Ph1/2(Out2) -> Mux/4
  TwoPtCon-1Ph1/1(Out1) -> Mux/3
  TwoPtCon-1Ph/2(Out2) -> Mux/2
  TwoPtCon-1Ph/1(Out1) -> Mux/1
  Mux/1 -> s05/1
  Iref/1 -> Demux1/1
  Iact/1 -> Demux/1
  Demux1/1 -> TwoPtCon-1Ph/1(In1)
  Demux1/2 -> TwoPtCon-1Ph1/1(In1)
  Demux1/3 -> TwoPtCon-1Ph2/1(In1)
  Demux/1 -> TwoPtCon-1Ph/2(In2)
  Demux/2 -> TwoPtCon-1Ph1/2(In2)
  Demux/3 -> TwoPtCon-1Ph2/2(In2)

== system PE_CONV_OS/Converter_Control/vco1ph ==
  note: Vpk
  Vp : Inport  OutDataType=sfix(16)  OutScaling=2^0
  w : Inport  Port=2  OutDataType=sfix(16)  OutScaling=2^0
  Th : Inport  Port=3  OutDataType=sfix(16)  OutScaling=2^0
  Clock : Clock
  Fcn : Fcn  Expr=u[1]*sin(u[2])
  Mux : Mux  Inputs=2
  Product : Product  OutDataType=sfix(16)  OutScaling=2^0
  Sum : Sum  Inputs=|++  OutDataType=sfix(16)  OutScaling=2^0
  y : Outport
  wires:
  Sum/1 -> Mux/2
  Th/1 -> Sum/2
  Product/1 -> Sum/1
  Clock/1 -> Product/2
  w/1 -> Product/1
  Fcn/1 -> y/1
  Mux/1 -> Fcn/1
  Vp/1 -> Mux/1

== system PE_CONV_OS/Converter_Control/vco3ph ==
  note: w
  note: Vpk
  note: -sin_wet
  note: cos_wet
  Vp : Inport  OutDataType=sfix(16)  OutScaling=2^0
  w : Inport  Port=2  OutDataType=sfix(16)  OutScaling=2^0
  -1 : Gain  Gain=-1  ParameterDataType=sfix(16)  ParameterScaling=2^0  OutDataType=sfix(16)  OutScaling=2^0
  Fcn : Fcn  Expr=u[1]*u[2]
  Fcn1 : Fcn  Expr=u[1]*(-u[2]-sqrt(3)*u[3])/2
  Fcn2 : Fcn  Expr=u[1]*(-u[2]+sqrt(3)*u[3])/2
  Inner Product : Subsystem
  Inner Product1 : Subsystem
  Mux : Mux  Inputs=3
  Mux1 : Mux  Inputs=3
  cos : Integrator  InitialCondition=1
  sin : Integrator
  y : Outport
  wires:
  w/1 -> Inner Product/1(in_1), Inner Product1/1(in_1)
  -1/1 -> sin/1
  Inner Product/1(out_1) -> -1/1
  Inner Product1/1(out_1) -> cos/1
  cos/1 -> Mux/2, Inner Product/2(in_2)
  sin/1 -> Mux/3, Inner Product1/2(in_2)
  Fcn/1 -> Mux1/1
  Fcn1/1 -> Mux1/2
  Fcn2/1 -> Mux1/3
  Mux/1 -> Fcn2/1, Fcn1/1, Fcn/1
  Vp/1 -> Mux/1
  Mux1/1 -> y/1
